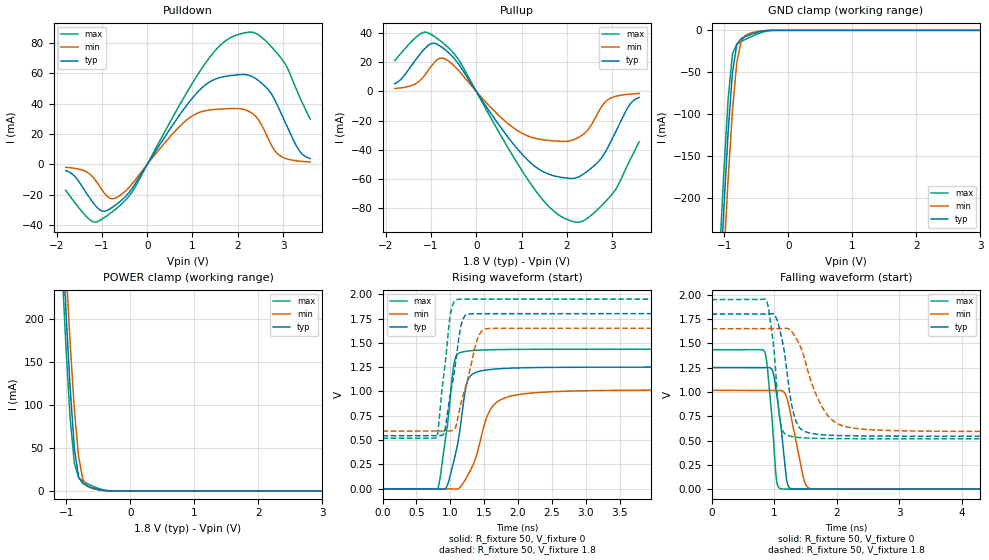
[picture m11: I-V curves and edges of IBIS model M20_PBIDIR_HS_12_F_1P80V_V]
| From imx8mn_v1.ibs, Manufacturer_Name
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[Model] M20_PBIDIR_HS_12_F_1P80V_V
Model_type I/O
Vinl  =  0.54
Vinh  =  1.26
Vmeas =  0.9
| Capacitance   typ   min   max
C_comp   1.53539775078e-12   1.44877555415e-12   1.57947525197e-12
| Variables   typ   min   max
[GND Clamp Reference]   0   0   0
[POWER Clamp Reference]   1.8   1.65   1.95
[Pulldown Reference]   0   0   0
[Pullup Reference]   1.8   1.65   1.95
[Temperature Range]   25   125   -40
[Voltage Range]   1.8   1.65   1.95
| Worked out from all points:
|   slope of the pulldown table from 0 to 0.27 V, typ, clamps not added: 21.3 ohm
|   slope of the pullup table from 0 to 0.27 V, typ, clamps not added: 21.4 ohm
|   GND clamp passes 1 mA (typ) near -0.41 V on its own axis
|   POWER clamp passes 1 mA (typ) near -0.45 V on its own axis
|   falling waveform, R_fixture 50, V_fixture 0: 20-80 % time 135ps typ, 188ps min, 105ps max; typ from 1.25 V to 0 V
|   falling waveform, R_fixture 50, V_fixture 1.8: 20-80 % time 182ps typ, 368ps min, 122ps max; typ from 1.8 V to 0.545 V
|   rising waveform, R_fixture 50, V_fixture 0: 20-80 % time 179ps typ, 285ps min, 145ps max; typ from 0 V to 1.25 V
|   rising waveform, R_fixture 50, V_fixture 1.8: 20-80 % time 165ps typ, 225ps min, 130ps max; typ from 0.545 V to 1.8 V
[GND Clamp]
| Voltage   I(typ)   I(min)   I(max)
-1.8V     -1.548A    -1.596A    -1.505A
-1.076V   -314.3mA   -373.2mA   -268.8mA
-1.009V   -212.8mA   -271.6mA   -169.3mA
-941.4mV  -121.4mA   -177.3mA   -82.2mA
-874.1mV  -50.48mA   -96.08mA   -28.29mA
-806.9mV  -17.11mA   -38.85mA   -16.39mA
-739.7mV  -9.89mA    -13.23mA   -13.32mA
-672.4mV  -7.354mA   -6.086mA   -10.75mA
-605.2mV  -5.342mA   -3.664mA   -8.302mA
-470.7mV  -2.022mA   -1.163mA   -3.923mA
-269mV    -32.89uA   -24.7uA    -158uA
3.6V      0A         0A         0A
[POWER Clamp]
| Voltage   I(typ)   I(min)   I(max)
-1.8V     1.548A     1.589A     1.509A
-1.076V   314.3mA    367.1mA    271.2mA
-1.009V   212.5mA    266.1mA    171.6mA
-941.4mV  120.5mA    172.9mA    85.18mA
-874.1mV  49.19mA    93.78mA    31.83mA
-806.9mV  15.58mA    38.69mA    15.29mA
-739.7mV  8.318mA    12.92mA    11.18mA
-672.4mV  5.835mA    5.348mA    8.546mA
-605.2mV  3.963mA    2.968mA    6.156mA
-470.7mV  1.193mA    886.9uA    2.247mA
-269mV    8.729uA    21.24uA    33.73uA
3.6V      0A         0A         0A
[Pulldown]
| Voltage   I(typ)   I(min)   I(max)
-1.8V     -4.07mA    -1.882mA   -17.02mA
-1.21V    -24.59mA   -7.922mA   -37.53mA
-874.1mV  -30.05mA   -21.26mA   -33.42mA
-605.2mV  -24.53mA   -20.45mA   -27.09mA
-269mV    -12.82mA   -10.29mA   -15mA
931mV     41.12mA    30.6mA     50.11mA
1.552V    56.59mA    36.27mA    76.44mA
2.002V    58.87mA    36.76mA    85.28mA
2.405V    56.24mA    31.42mA    86.03mA
2.876V    38.89mA    7.059mA    72.82mA
3.347V    9.502mA    2.185mA    45.74mA
3.6V      3.859mA    1.564mA    29.89mA
[Pullup]
| Voltage   I(typ)   I(min)   I(max)
-1.8V     5.253mA    1.975mA    21.1mA
-1.21V    26.7mA     8.395mA    39.94mA
-874.1mV  32.48mA    21.41mA    36.47mA
-403.4mV  19.29mA    14.79mA    22.37mA
496.6mV   -22.74mA   -16.4mA    -27.64mA
1.117V    -46.43mA   -30.23mA   -59.35mA
1.614V    -56.83mA   -33.63mA   -79.19mA
2.069V    -59.6mA    -33.89mA   -88.46mA
2.405V    -55.88mA   -28.44mA   -87.92mA
2.943V    -36.28mA   -5.018mA   -72.51mA
3.347V    -11.17mA   -2.008mA   -50.26mA
3.6V      -4.164mA   -1.438mA   -34.59mA
[Ramp]
dV/dt_r   0.750384/0.178824n  0.609482/0.284575n  0.860548/0.144545n
dV/dt_f   0.753164/0.181738n  0.634351/0.367645n  0.858826/0.121637n
R_load = 50
[Falling Waveform]
R_fixture = 50
V_fixture = 0
V_fixture_min = 0
V_fixture_max = 0
| Time   V(typ)   V(min)   V(max)
0s        1.251V     1.016V     1.434V
846.9ps   1.251V     1.016V     1.418V
892.4ps   1.251V     1.016V     1.255V
974ps     1.219V     1.016V     671.4mV
1.045ns   955.1mV    1.016V     68.44mV
1.194ns   124.6mV    957.3mV    1.086mV
1.268ns   7.229mV    760.5mV    668.3uV
1.495ns   748.9uV    64.87mV    426.5uV
1.741ns   360.4uV    884.1uV    163.9uV
333.3ns   59.13nV    328.3nV    41.44nV
[Falling Waveform]
R_fixture = 50
V_fixture = 1.8
V_fixture_min = 1.65
V_fixture_max = 1.95
| Time   V(typ)   V(min)   V(max)
0s        1.8V       1.65V      1.95V
864.4ps   1.8V       1.65V      1.952V
1.005ns   1.796V     1.65V      1.39V
1.083ns   1.661V     1.65V      766.1mV
1.151ns   1.465V     1.652V     585.6mV
1.271ns   903mV      1.629V     542.8mV
1.375ns   663.5mV    1.526V     532.3mV
1.909ns   554.4mV    722.7mV    520.1mV
5.467ns   544.7mV    592.9mV    518.7mV
333.3ns   544.7mV    592.7mV    518.6mV
[Rising Waveform]
R_fixture = 50
V_fixture = 0
V_fixture_min = 0
V_fixture_max = 0
| Time   V(typ)   V(min)   V(max)
0s        43.75nV    327.8nV    36.24nV
816.3ps   -209.3uV   24.73uV    7.94mV
947.1ps   21.22mV    -105.7uV   597.2mV
1.042ns   254.4mV    -2.244mV   1.229V
1.102ns   434.1mV    -3.653mV   1.379V
1.221ns   1.007V     92.16mV    1.412V
1.293ns   1.156V     184.1mV    1.419V
1.599ns   1.227V     821.1mV    1.429V
1.988ns   1.242V     965.9mV    1.433V
333.3ns   1.251V     1.016V     1.434V
[Rising Waveform]
R_fixture = 50
V_fixture = 1.8
V_fixture_min = 1.65
V_fixture_max = 1.95
| Time   V(typ)   V(min)   V(max)
0s        544.7mV    592.7mV    518.6mV
800.1ps   544.7mV    592.7mV    531.7mV
822.9ps   544.5mV    592.7mV    613mV
912.1ps   576.3mV    592.7mV    1.211V
1.004ns   980.5mV    594.3mV    1.805V
1.083ns   1.316V     642.4mV    1.941V
1.183ns   1.735V     944.1mV    1.949V
1.437ns   1.799V     1.595V     1.95V
1.794ns   1.8V       1.649V     1.95V
333.3ns   1.8V       1.65V      1.95V
[Add Submodel]
| Submodel Name Mode
M20_PBIDIR_HS_12_F_1P80V_T_V All
